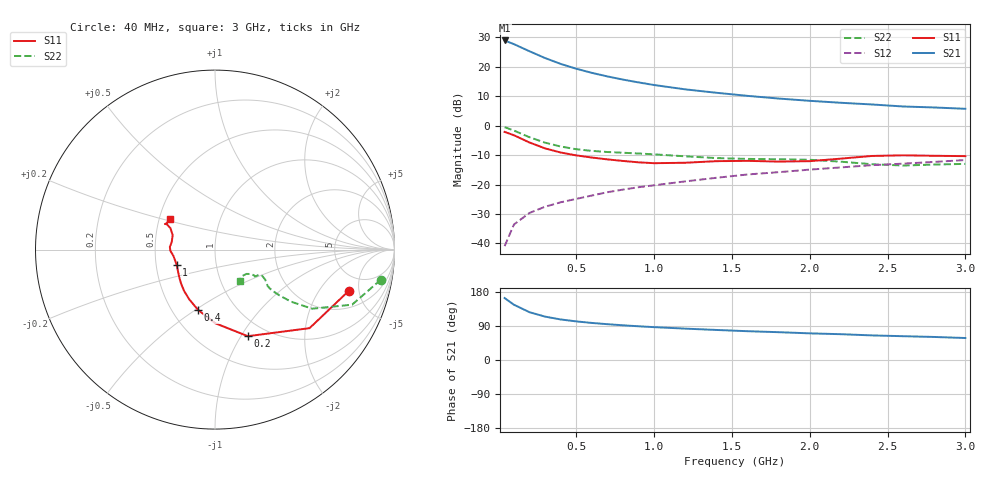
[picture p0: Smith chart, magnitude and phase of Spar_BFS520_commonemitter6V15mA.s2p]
! Filename:  BFS520J.S2P  Version:  4.0
! NXP part #: BFS520  Date: Jun 1994
! Bias condition: Vce=6V, Ic=15mA
#  MHz  S  MA  R  50
! Freq  S11  S21  S12  S22  !GUM [dB]
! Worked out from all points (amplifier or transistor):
!   21 points, 40 MHz to 3 GHz, reference 50 ohm
!   highest |S21| = 28.9 dB at 40 MHz (marker M1)
!   |S21| within 3 dB of that: start of sweep to 172.3 MHz
!   unconditionally stable (mu >= 1): 792.7 MHz to end of sweep
!   at 300 MHz: K = 0.71, MSG = 25.2 dB, |S12| = -27.5 dB
!   at 1 GHz: K = 1.06, MAG = 15.5 dB, |S12| = -20.3 dB
!   at 3 GHz: K = 1.06, MAG = 7.3 dB, |S12| = -11.7 dB
!   lowest NFmin = 1.30 dB at 500 MHz
!   S11 on the Smith chart (normalised r, x): 40 MHz: 3.36, -3.93; 200 MHz: 0.82, -1.07; 400 MHz: 0.67, -0.51; 1 GHz: 0.64, -0.12; 3 GHz: 0.57, +0.22
40  0.781 -17.0  27.78 163.5  0.009 81.3  0.939 -10.3
100  0.685 -39.7  24.05 145.8  0.021 70.7  0.823 -21.9
200  0.516 -69.2  18.2 126.1  0.033 63.5  0.634 -31.3
300  0.41 -89.9  13.96 114.5  0.042 62.3  0.513 -34.4
400  0.349 -105.7  11.12 107.0  0.05 63.3  0.441 -35.4
500  0.312 -117.4  9.205 101.9  0.057 64.9  0.397 -35.6
600  0.287 -127.0  7.841 97.8  0.065 66.2  0.372 -35.3
700  0.267 -135.2  6.821 94.5  0.074 67.5  0.356 -34.6
800  0.251 -142.7  6.025 91.6  0.082 68.7  0.346 -33.4
900  0.238 -150.3  5.396 89.0  0.09 69.4  0.336 -32.1
1000  0.23 -157.9  4.874 86.7  0.097 70.1  0.325 -30.8
1200  0.234 -171.1  4.115 82.8  0.113 70.9  0.301 -29.1
1400  0.249 -178.6  3.601 79.3  0.13 71.7  0.281 -30.1
1600  0.252 176.6  3.191 76.0  0.148 71.3  0.272 -33.1
1800  0.245 170.7  2.874 73.4  0.162 71.8  0.268 -34.0
2000  0.249 161.2  2.629 70.3  0.179 71.6  0.263 -33.5
2200  0.275 154.4  2.436 68.1  0.195 71.6  0.244 -33.8
2400  0.305 152.1  2.279 64.9  0.213 71.2  0.221 -37.8
2600  0.313 153.0  2.108 62.8  0.226 70.3  0.21 -45.2
2800  0.307 151.3  2.027 60.8  0.242 70.5  0.218 -50.4
3000  0.303 145.6  1.926 58.0  0.26 69.8  0.224 -52.0
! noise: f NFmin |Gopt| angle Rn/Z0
500  1.3  0.192  26  0.23
900  1.45  0.158  56  0.23
2000  2.05  0.202  175  0.18
